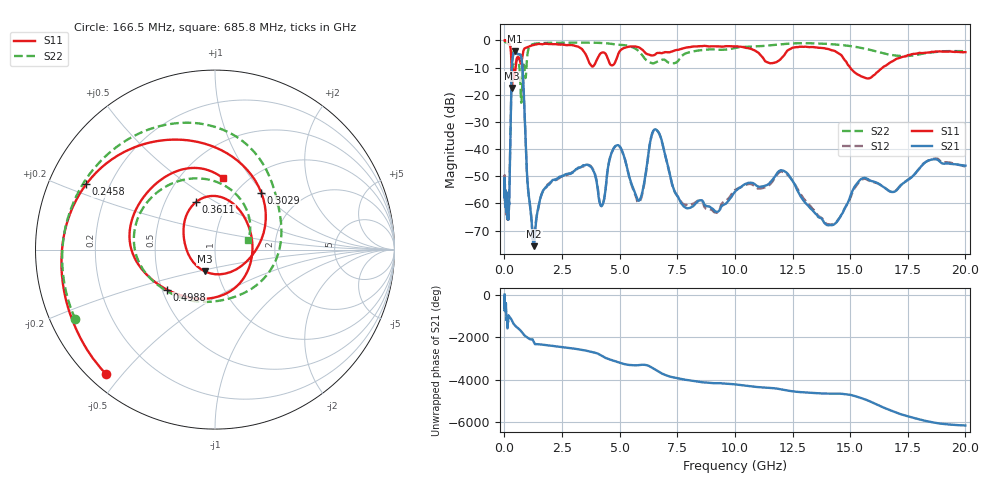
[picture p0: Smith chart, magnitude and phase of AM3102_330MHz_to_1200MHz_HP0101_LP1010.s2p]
! Date/Time: Tue, Sep 11, 2018 5:14 PM
! Network Analyzer: Agilent Technologies E8362B Rev: A.07.50.63
! Sweep from 0.010 to 20.000 GHz, 1601 Points, Sweep Type: LOG
! Power Supply: 4.949 V, 0.001 A
# Hz S DB R 50
!freq MagS11 AngS11 MagS21 AngS21 MagS12 AngS12 MagS22 AngS22
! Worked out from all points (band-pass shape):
!   1601 points, 10 MHz to 20 GHz, reference 50 ohm
!   highest |S21| = -3.95 dB at 460.1 MHz (marker M1); lowest = -75.7 dB at 1.284 GHz (marker M2)
!   |S21| within 3 dB of the highest: 349.3 MHz to 748.9 MHz (399.6 MHz wide, 72.8 % of centre)
!   lowest |S11| = -17.5 dB at 331.5 MHz (marker M3), VSWR 1.31, Z = 43.5 - j10.8 ohm
!   |S11| at or under -10 dB: 309.6 MHz to 488.8 MHz (179.1 MHz wide, 44.9 % of centre); 15 GHz to 16.41 GHz (1.403 GHz wide, 8.93 % of centre)
!   |S22| runs from -22.9 to -0.3 dB; largest |S21 - S12| = 0.011
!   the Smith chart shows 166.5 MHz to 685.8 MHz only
!   S11 on the Smith chart (normalised r, x): 166.5 MHz: 0.05, -0.45; 245.8 MHz: 0.11, +0.24; 302.9 MHz: 1.28, +0.97; 361.1 MHz: 0.71, +0.41; 498.8 MHz: 0.53, -0.27; 685.8 MHz: 0.79, +0.74
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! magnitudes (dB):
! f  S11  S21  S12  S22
! 10 MHz  0.0  -52.3  -49.8  -0.3
! 35.55 MHz  0.0  -58.8  -58.7  -0.5
! 126.4 MHz  -0.4  -64.5  -65.2  -1.0
! 166.5 MHz  -0.7  -64.8  -65.7  -1.2
! 245.8 MHz  -1.9  -42.6  -42.7  -1.8
! 302.9 MHz  -7.8  -16.9  -16.9  -3.7
! 331.5 MHz  -17.5  -9.1  -9.1  -6.4
! 361.1 MHz  -10.9  -6.2  -6.3  -8.6
! 447.2 MHz  -12.5  -4.0  -4.0  -10.2
! 460.1 MHz  -11.8  -4.0  -4.0  -9.7
! 498.8 MHz  -9.2  -4.1  -4.2  -8.2
! 685.8 MHz  -8.0  -5.1  -5.2  -14.3
! 1.284 GHz  -1.6  -75.7  -74.1  -1.2
! 1.59 GHz  -1.4  -57.2  -57.1  -0.9
! 4.23 GHz  -4.5  -60.9  -60.9  -0.9
! 4.878 GHz  -6.5  -38.6  -38.7  -1.5
! 5.652 GHz  -2.2  -55.9  -56.4  -2.9
! 6.58 GHz  -4.9  -32.8  -32.9  -8.0
! 7.958 GHz  -2.5  -61.8  -60.8  -4.5
! 12.03 GHz  -6.4  -47.8  -48.3  -1.4
! 14.14 GHz  -3.4  -68.0  -67.9  -1.3
! 20 GHz  -4.3  -46.1  -46.5  -3.9
